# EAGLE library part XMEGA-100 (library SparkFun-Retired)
Atmel XMega uC Not in catalog
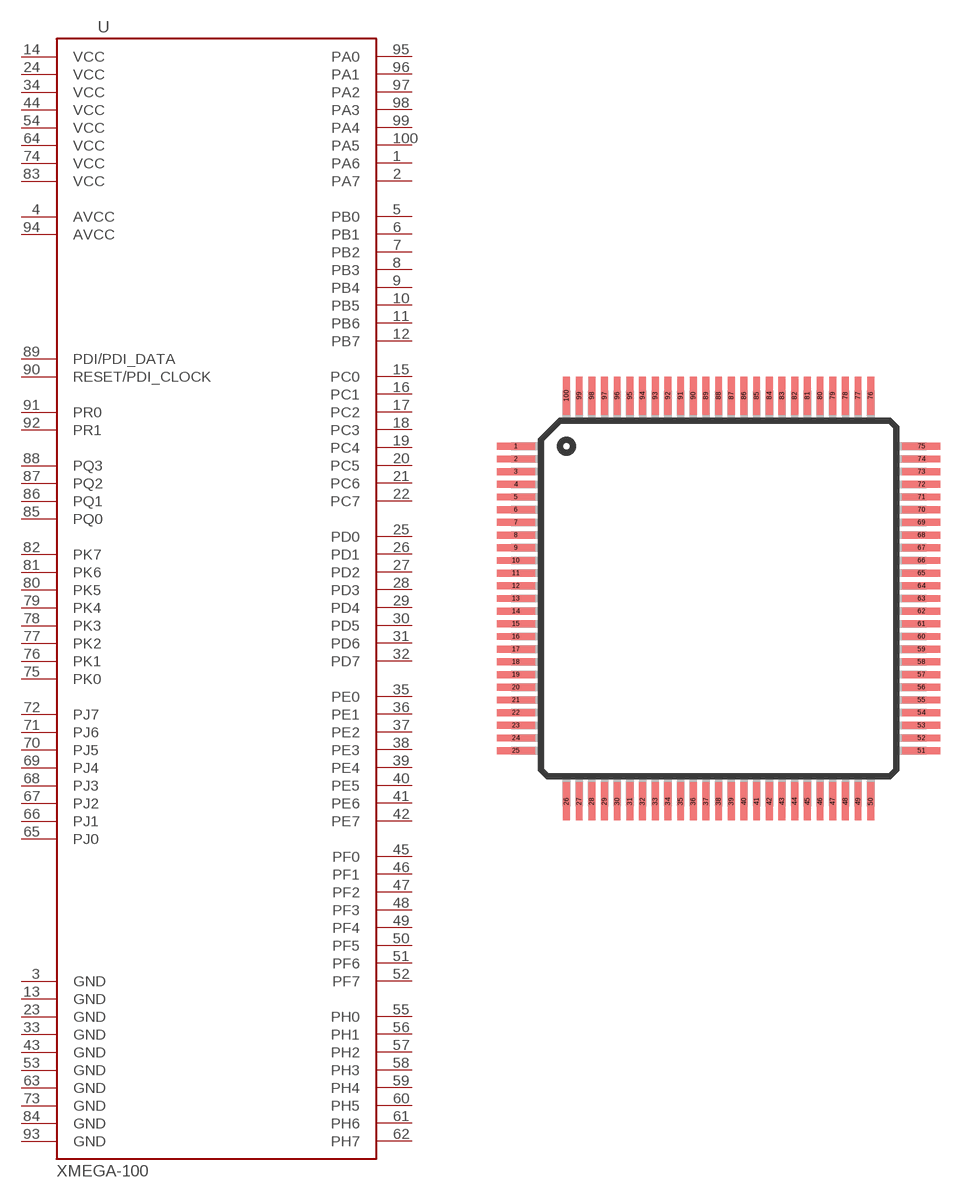
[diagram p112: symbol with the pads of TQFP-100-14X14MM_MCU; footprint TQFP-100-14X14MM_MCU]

Designator prefix -

## XMEGA-100SMD  [TQFP-100-14X14MM_MCU]
1  PA6
2  PA7
3  GND
4  AVCC
5  PB0
6  PB1
7  PB2
8  PB3
9  PB4
10  PB5
11  PB6
12  PB7
13  GND
14  VCC
15  PC0
16  PC1
17  PC2
18  PC3
19  PC4
20  PC5
21  PC6
22  PC7
23  GND
24  VCC
25  PD0
26  PD1
27  PD2
28  PD3
29  PD4
30  PD5
31  PD6
32  PD7
33  GND
34  VCC
35  PE0
36  PE1
37  PE2
38  PE3
39  PE4
40  PE5
41  PE6
42  PE7
43  GND
44  VCC
45  PF0
46  PF1
47  PF2
48  PF3
49  PF4
50  PF5
51  PF6
52  PF7
53  GND
54  VCC
55  PH0
56  PH1
57  PH2
58  PH3
59  PH4
60  PH5
61  PH6
62  PH7
63  GND
64  VCC
65  PJ0
66  PJ1
67  PJ2
68  PJ3
69  PJ4
70  PJ5
71  PJ6
72  PJ7
73  GND
74  VCC
75  PK0
76  PK1
77  PK2
78  PK3
79  PK4
80  PK5
81  PK6
82  PK7
83  VCC
84  GND
85  PQ0
86  PQ1
87  PQ2
88  PQ3
89  PDI/PDI_DATA
90  RESET/PDI_CLOCK
91  PR0
92  PR1
93  GND
94  AVCC
95  PA0
96  PA1
97  PA2
98  PA3
99  PA4
100  PA5

## Footprint TQFP-100-14X14MM_MCU (pad centres in mm)
smd 1.5 x 0.27: 1 -8,6; 2 -8,5.5; 3 -8,5; 4 -8,4.5; 5 -8,4; 6 -8,3.5; 7 -8,3; 8 -8,2.5; 9 -8,2; 10 -8,1.5; 11 -8,1; 12 -8,0.5; 13 -8,0; 14 -8,-0.5; 15 -8,-1; 16 -8,-1.5; 17 -8,-2; 18 -8,-2.5; 19 -8,-3; 20 -8,-3.5; 21 -8,-4; 22 -8,-4.5; 23 -8,-5; 24 -8,-5.5; 25 -8,-6; 51 8,-6; 52 8,-5.5; 53 8,-5; 54 8,-4.5; 55 8,-4; 56 8,-3.5; 57 8,-3; 58 8,-2.5; 59 8,-2; 60 8,-1.5; 61 8,-1; 62 8,-0.5; 63 8,0; 64 8,0.5; 65 8,1; 66 8,1.5; 67 8,2; 68 8,2.5; 69 8,3; 70 8,3.5; 71 8,4; 72 8,4.5; 73 8,5; 74 8,5.5; 75 8,6
smd 0.27 x 1.5: 26 -6,-8; 27 -5.5,-8; 28 -5,-8; 29 -4.5,-8; 30 -4,-8; 31 -3.5,-8; 32 -3,-8; 33 -2.5,-8; 34 -2,-8; 35 -1.5,-8; 36 -1,-8; 37 -0.5,-8; 38 0,-8; 39 0.5,-8; 40 1,-8; 41 1.5,-8; 42 2,-8; 43 2.5,-8; 44 3,-8; 45 3.5,-8; 46 4,-8; 47 4.5,-8; 48 5,-8; 49 5.5,-8; 50 6,-8; 76 6,8; 77 5.5,8; 78 5,8; 79 4.5,8; 80 4,8; 81 3.5,8; 82 3,8; 83 2.5,8; 84 2,8; 85 1.5,8; 86 1,8; 87 0.5,8; 88 0,8; 89 -0.5,8; 90 -1,8; 91 -1.5,8; 92 -2,8; 93 -2.5,8; 94 -3,8; 95 -3.5,8; 96 -4,8; 97 -4.5,8; 98 -5,8; 99 -5.5,8; 100 -6,8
